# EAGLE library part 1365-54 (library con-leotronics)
DUAL ROW STRAIGHT HEADER 1364 SERIES. 1.27mm x 1.27mm. Without Fixing Post. SMT Source: http://www.leotronics.co.uk/Conexcon/Data%20Sheets/sec.%20A/1364ing.pdf
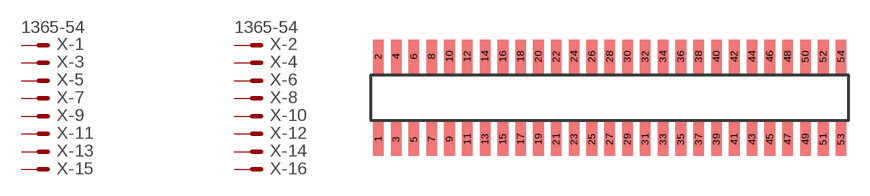
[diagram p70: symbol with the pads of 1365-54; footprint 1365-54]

Designator prefix X; gates -1=MVAL -2=MVAL -3=M -4=M -5=M -6=M -7=M -8=M -9=M -10=M -11=M -12=M -13=M -14=M -15=M -16=M -17=M -18=M -19=M -20=M -21=M -22=M -23=M -24=M -25=M -26=M -27=M -28=M -29=M -30=M -31=M -32=M -33=M -34=M -35=M -36=M -37=M -38=M -39=M -40=M -41=M -42=M -43=M -44=M -45=M -46=M -47=M -48=M -49=M -50=M -51=M -52=M -53=M -54=M

## 1365-54 (OC_FARNELL: unknown; OC_NEWARK: unknown)  [1365-54]
1  -1:S  pas
2  -2:S  pas
3  -3:S  pas
4  -4:S  pas
5  -5:S  pas
6  -6:S  pas
7  -7:S  pas
8  -8:S  pas
9  -9:S  pas
10  -10:S  pas
11  -11:S  pas
12  -12:S  pas
13  -13:S  pas
14  -14:S  pas
15  -15:S  pas
16  -16:S  pas
17  -17:S  pas
18  -18:S  pas
19  -19:S  pas
20  -20:S  pas
21  -21:S  pas
22  -22:S  pas
23  -23:S  pas
24  -24:S  pas
25  -25:S  pas
26  -26:S  pas
27  -27:S  pas
28  -28:S  pas
29  -29:S  pas
30  -30:S  pas
31  -31:S  pas
32  -32:S  pas
33  -33:S  pas
34  -34:S  pas
35  -35:S  pas
36  -36:S  pas
37  -37:S  pas
38  -38:S  pas
39  -39:S  pas
40  -40:S  pas
41  -41:S  pas
42  -42:S  pas
43  -43:S  pas
44  -44:S  pas
45  -45:S  pas
46  -46:S  pas
47  -47:S  pas
48  -48:S  pas
49  -49:S  pas
50  -50:S  pas
51  -51:S  pas
52  -52:S  pas
53  -53:S  pas
54  -54:S  pas

## Footprint 1365-54 (pad centres in mm)
DUAL ROW STRAIGHT HEADER 1364 SERIES. 1.27mm x 1.27mm. Without Fixing Post. SMT Source: http://www.leotronics.co.uk/Conexcon/Data%20Sheets/sec.%20A/1364ing.pdf
smd 0.76 x 2.4: 1 -16.51,-2.95; 2 -16.51,2.95; 3 -15.24,-2.95; 4 -15.24,2.95; 5 -13.97,-2.95; 6 -13.97,2.95; 7 -12.7,-2.95; 8 -12.7,2.95; 9 -11.43,-2.95; 10 -11.43,2.95; 11 -10.16,-2.95; 12 -10.16,2.95; 13 -8.89,-2.95; 14 -8.89,2.95; 15 -7.62,-2.95; 16 -7.62,2.95; 17 -6.35,-2.95; 18 -6.35,2.95; 19 -5.08,-2.95; 20 -5.08,2.95; 21 -3.81,-2.95; 22 -3.81,2.95; 23 -2.54,-2.95; 24 -2.54,2.95; 25 -1.27,-2.95; 26 -1.27,2.95; 27 0,-2.95; 28 0,2.95; 29 1.27,-2.95; 30 1.27,2.95; 31 2.54,-2.95; 32 2.54,2.95; 33 3.81,-2.95; 34 3.81,2.95; 35 5.08,-2.95; 36 5.08,2.95; 37 6.35,-2.95; 38 6.35,2.95; 39 7.62,-2.95; 40 7.62,2.95; 41 8.89,-2.95; 42 8.89,2.95; 43 10.16,-2.95; 44 10.16,2.95; 45 11.43,-2.95; 46 11.43,2.95; 47 12.7,-2.95; 48 12.7,2.95; 49 13.97,-2.95; 50 13.97,2.95; 51 15.24,-2.95; 52 15.24,2.95; 53 16.51,-2.95; 54 16.51,2.95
